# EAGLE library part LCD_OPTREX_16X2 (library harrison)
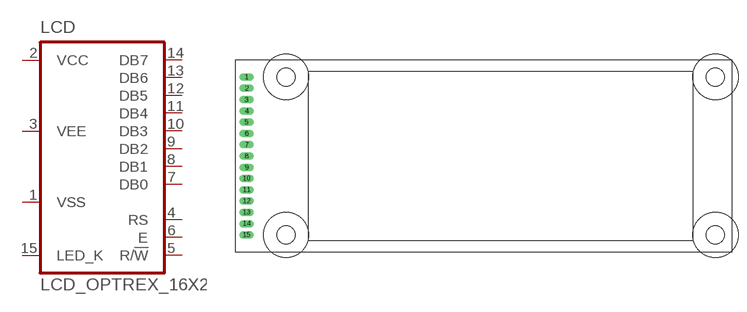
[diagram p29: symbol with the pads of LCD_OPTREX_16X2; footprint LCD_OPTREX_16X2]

Designator prefix LCD

## LCD_OPTREX_16X2  [LCD_OPTREX_16X2]
1  VSS  pwr
2  VCC  pwr
3  VEE  pwr
4  RS  in
5  R/!W!  in
6  E  in
7  DB0  in
8  DB1  in
9  DB2  in
10  DB3  in
11  DB4  in
12  DB5  in
13  DB6  in
14  DB7  in
15  LED_K  pas

## Footprint LCD_OPTREX_16X2 (pad centres in mm)
drill 0.8 long: 1 2,31; 2 2,29; 3 2,27; 4 2,25; 5 2,23; 6 2,21; 7 2,19; 8 2,17; 9 2,15; 10 2,13; 11 2,11; 12 2,9; 13 2,7; 14 2,5; 15 2,3
hole 3.2 at 9,3
hole 3.2 at 9,31
hole 3.2 at 85,31
hole 3.2 at 85,3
